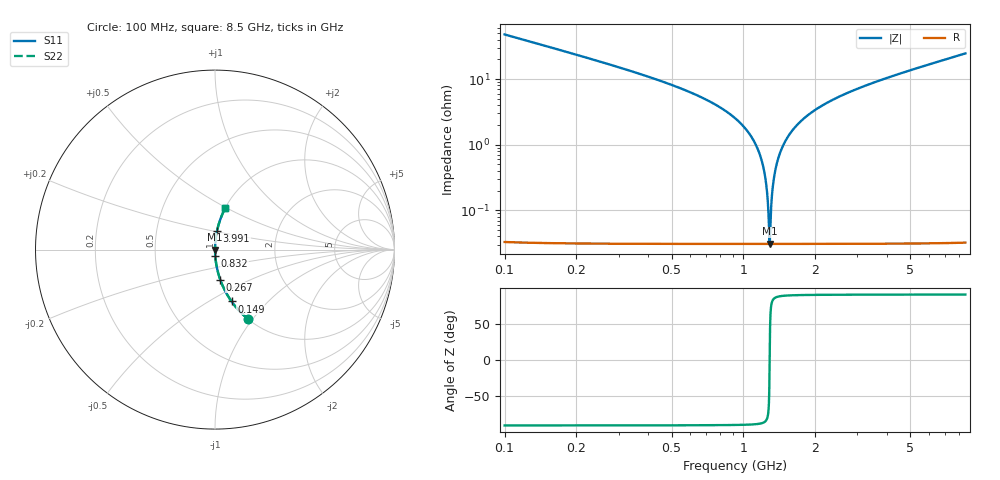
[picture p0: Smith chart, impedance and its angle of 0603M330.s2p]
! Created Wed Apr 18 16:47:35 2012
# hz S ma R 50
! 2 Port Network Data from SP1.SP block
! freq  magS11  angS11  magS21  angS21  magS12  angS12  magS22  angS22
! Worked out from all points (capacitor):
!   8401 points, 100 MHz to 8.5 GHz, reference 50 ohm
!   read as one part in series: C = 33.1 pF near 142 MHz
!   lowest |Z| = 30.9 mohm at 1.288 GHz (marker M1)
!   series resonance near 1.288 GHz, so ESL is about 460 pH
!   S11 on the Smith chart (normalised r, x): 100 MHz: 1.00, -0.95; 149 MHz: 1.00, -0.64; 267 MHz: 1.00, -0.34; 832 MHz: 1.00, -0.07; 3.991 GHz: 1.00, +0.21; 8.5 GHz: 1.00, +0.49
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1e8  0.4306 -64.5  0.9023 25.5  0.9023 25.5  0.4306 -64.5
1.49e8  0.3029 -72.3  0.9527 17.6  0.9527 17.6  0.3029 -72.3
2.67e8  0.1695 -80.1  0.9852 9.8  0.9852 9.8  0.1695 -80.1
8.32e8  0.03359 -87.6  0.9991 1.9  0.9991 1.9  0.03359 -87.6
1.019e9  0.0176 -88.0  0.9995 1.0  0.9995 1.0  0.0176 -88.0
1.142e9  0.008973 -87.5  0.9997 0.5  0.9997 0.5  0.008973 -87.5
1.208e9  0.00477 -86.0  0.9997 0.3  0.9997 0.3  0.00477 -86.0
1.231e9  0.003366 -84.6  0.9997 0.2  0.9997 0.2  0.003366 -84.6
1.26e9  0.001643 -79.1  0.9997 0.1  0.9997 0.1  0.001643 -79.1
1.288e9  0.0003089 4.7  0.9997 -0.0  0.9997 -0.0  0.0003089 4.7
1.314e9  0.001547 78.4  0.9997 -0.1  0.9997 -0.1  0.001547 78.4
1.348e9  0.003436 84.7  0.9997 -0.2  0.9997 -0.2  0.003436 84.7
1.382e9  0.005293 86.4  0.9997 -0.3  0.9997 -0.3  0.005293 86.4
1.5e9  0.01144 87.8  0.9996 -0.7  0.9996 -0.7  0.01144 87.8
1.687e9  0.0204 88.0  0.9995 -1.2  0.9995 -1.2  0.0204 88.0
1.967e9  0.03256 87.6  0.9992 -1.9  0.9992 -1.9  0.03256 87.6
2.9e9  0.0674 85.9  0.9974 -3.9  0.9974 -3.9  0.0674 85.9
3.991e9  0.1034 83.9  0.9943 -5.9  0.9943 -5.9  0.1034 83.9
4.3e9  0.1131 83.3  0.9933 -6.5  0.9933 -6.5  0.1131 83.3
5.7e9  0.156 80.9  0.9874 -9.0  0.9874 -9.0  0.156 80.9
7.1e9  0.1976 78.5  0.98 -11.4  0.98 -11.4  0.1976 78.5
8.5e9  0.2384 76.1  0.9709 -13.8  0.9709 -13.8  0.2384 76.1
